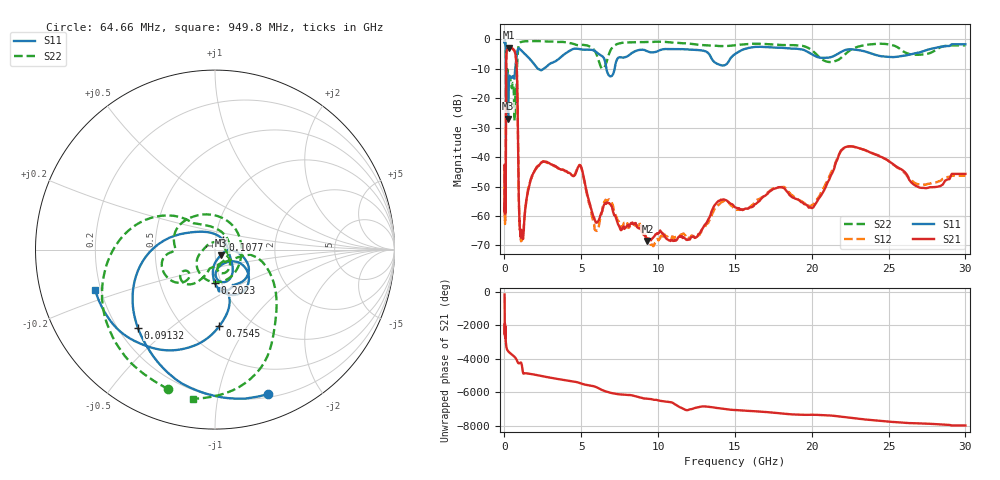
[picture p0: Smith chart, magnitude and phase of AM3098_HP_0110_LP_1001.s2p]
! Date/Time: Thu, Feb 28, 2019 8:37 AM
! Network Analyzer: Agilent Technologies E8364B Rev: A.07.50.67
! Sweep from 0.010 to 30.000 GHz, 1601 Points, Sweep Type: LOG
! Power Supply: 5.022 V, 0.002 A
# Hz S DB R 50
!freq MagS11 AngS11 MagS21 AngS21 MagS12 AngS12 MagS22 AngS22
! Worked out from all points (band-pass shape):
!   1601 points, 10 MHz to 30 GHz, reference 50 ohm
!   highest |S21| = -2.80 dB at 302 MHz (marker M1); lowest = -68.5 dB at 9.302 GHz (marker M2)
!   |S21| within 3 dB of the highest: 118.1 MHz to 735.9 MHz (617.7 MHz wide, 145 % of centre)
!   lowest |S11| = -27.0 dB at 238.7 MHz (marker M3), VSWR 1.09, Z = 53.3 - j3.25 ohm
!   |S11| at or under -10 dB: 99.91 MHz to 701.9 MHz (602 MHz wide, 150 % of centre); 2.191 GHz to 2.546 GHz (354.7 MHz wide, 15 % of centre); 6.637 GHz to 7.168 GHz (530.8 MHz wide, 7.69 % of centre)
!   |S22| runs from -27.6 to -0.5 dB; largest |S21 - S12| = 0.014
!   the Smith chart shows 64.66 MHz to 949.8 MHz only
!   S11 on the Smith chart (normalised r, x): 64.66 MHz: 0.23, -1.41; 91.32 MHz: 0.28, -0.39; 107.7 MHz: 1.09, +0.12; 202.3 MHz: 0.93, -0.36; 754.5 MHz: 0.72, -0.75; 949.8 MHz: 0.18, -0.16
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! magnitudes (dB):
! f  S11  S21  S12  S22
! 10 MHz  -0.4  -42.6  -43.3  -0.6
! 38.04 MHz  -0.5  -58.5  -60.4  -0.9
! 64.66 MHz  -1.3  -52.5  -52.7  -1.7
! 91.32 MHz  -4.3  -36.8  -37.1  -4.7
! 107.7 MHz  -23.0  -9.2  -9.2  -21.7
! 144.7 MHz  -18.9  -3.8  -3.8  -14.1
! 202.3 MHz  -14.6  -3.2  -3.2  -10.8
! 238.7 MHz  -27.0  -2.9  -2.9  -12.6
! 302 MHz  -14.1  -2.8  -2.7  -12.5
! 550.5 MHz  -12.5  -3.3  -3.3  -14.8
! 754.5 MHz  -7.4  -6.6  -6.6  -21.3
! 833.9 MHz  -4.2  -15.9  -15.9  -7.6
! 949.8 MHz  -3.0  -58.3  -57.8  -1.5
! 1.208 GHz  -4.3  -67.8  -64.5  -0.7
! 2.084 GHz  -9.4  -43.4  -43.9  -0.6
! 4.903 GHz  -3.3  -42.6  -42.7  -2.0
! 5.9 GHz  -4.0  -61.5  -64.7  -4.1
! 7.926 GHz  -5.9  -63.8  -62.5  -1.0
! 9.302 GHz  -4.1  -68.5  -67.7  -0.9
! 19.9 GHz  -4.7  -57.1  -56.7  -3.2
! 22.67 GHz  -3.4  -36.4  -36.4  -3.1
! 30 GHz  -1.6  -45.7  -46.3  -2.0
